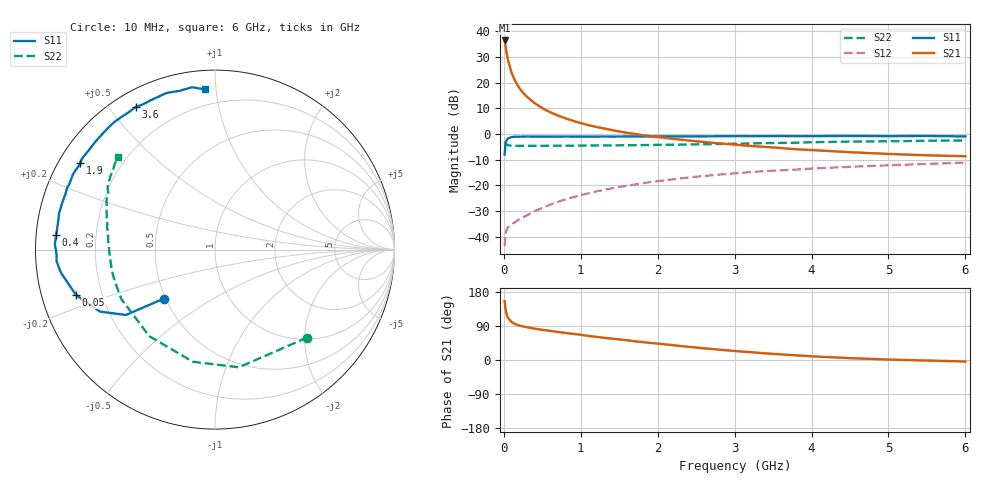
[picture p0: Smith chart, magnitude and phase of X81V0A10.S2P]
! SIEMENS Small Signal Semiconductors
! BFP136W
! Si NPN RF Bipolar Junction Transistor in SOT343
! VCE = 1 V  IC = 100 mA
! Common Emitter S-Parameters:  September  1994
# GHz  S  MA  R  50
!  f  S11  S21  S12  S22
! GHz  MAG  ANG  MAG  ANG  MAG  ANG  MAG  ANG
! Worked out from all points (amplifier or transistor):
!   40 points, 10 MHz to 6 GHz, reference 50 ohm
!   highest |S21| = 36.5 dB at 10 MHz (marker M1)
!   |S21| within 3 dB of that: start of sweep to 25.97 MHz
!   unconditionally stable (mu >= 1): 418.6 MHz to 3.487 GHz; 3.665 GHz to 4.049 GHz; 4.897 GHz to 5.104 GHz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
!   at 200 MHz: K = 0.75, MSG = 25.6 dB, |S12| = -33.2 dB
!   at 1.5 GHz: K = 1.14, MAG = 8.6 dB, |S12| = -20.7 dB
!   at 6 GHz: K = 1.03, MAG = 0.1 dB, |S12| = -11.2 dB
!   S11 on the Smith chart (normalised r, x): 10 MHz: 0.49, -0.32; 50 MHz: 0.10, -0.16; 400 MHz: 0.06, +0.05; 1.9 GHz: 0.06, +0.29; 3.6 GHz: 0.06, +0.59; 6 GHz: 0.10, +0.93
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0.01  0.3959 -136.3  66.48 155.4  0.0065 63.1  0.7095 -43.7
0.02  0.6148 -143.7  53.76 137.0  0.0104 49.5  0.6691 -78.5
0.03  0.727 -151.6  43.02 125.3  0.0126 43.3  0.6369 -101.2
0.05  0.8147 -161.9  29.22 112.5  0.015 33.1  0.6055 -127.3
0.1  0.8687 -171.6  15.64 100.0  0.0173 33.8  0.5899 -152.1
0.15  0.8854 -175.9  10.54 94.5  0.0193 38.7  0.5857 -161.6
0.2  0.883 -178.3  7.889 91.0  0.0218 41.6  0.5855 -166.6
0.25  0.8883 179.5  6.355 88.4  0.0238 46.3  0.5865 -169.7
0.3  0.8925 178.1  5.31 86.5  0.0259 48.9  0.5851 -171.9
0.4  0.889 174.8  4.001 82.7  0.0314 53.2  0.5866 -174.9
0.5  0.8872 172.7  3.188 79.6  0.0361 56.4  0.5872 -177.1
0.7  0.889 168.5  2.298 73.9  0.0472 60.6  0.5897 -179.7
0.9  0.8902 165.0  1.806 68.9  0.0583 61.5  0.5917 177.9
1.1  0.8893 160.8  1.484 63.4  0.0698 61.8  0.5947 176.3
1.5  0.8918 154.3  1.115 54.3  0.0925 60.4  0.6002 172.8
1.9  0.8937 147.2  0.909 45.2  0.1148 57.4  0.6091 169.5
2.2  0.8949 142.1  0.804 39.0  0.1308 54.7  0.6161 166.8
3.2  0.9041 125.1  0.585 20.7  0.1799 44.4  0.6528 157.5
3.6  0.9096 118.9  0.532 14.9  0.1963 40.2  0.6694 153.8
4.5  0.9135 107.2  0.441 4.9  0.2292 31.5  0.7092 145.7
5.5  0.9137 98.1  0.384 -1.4  0.2609 23.5  0.7369 139.0
6  0.8946 93.7  0.368 -3.9  0.2766 19.1  0.7473 136.2
